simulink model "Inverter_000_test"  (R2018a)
settings: Solver=FixedStepDiscrete  StartTime=0.0  StopTime=inf  RelTol=1e-3  EnableMultiTasking=on
PreLoadFcn:
  | Sample_Time
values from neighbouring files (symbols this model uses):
  Tcontrol = 5e-5     *2    (= 0.0001)    [Sample_Time.m]
undefined symbols (not defined in the file or in its folder): A, ADCIN0, ADCIN1, ADCINA0, ADCINB0, bit, Compare, conversion, DCAEVT1, DCAEVT1FILT, Digital, Down, ended, Event, Filtered, GPTRIP1SEL, GPTRIP2SEL, input, Module, of, Single, start, Trip, TZ1, TZ2, Up, version, Zone
libraries: tiiqmathlib x19, c2837xDlib x6, c2802xlib x5, simulink x4, etargetslib x4, c28xdmclib x1

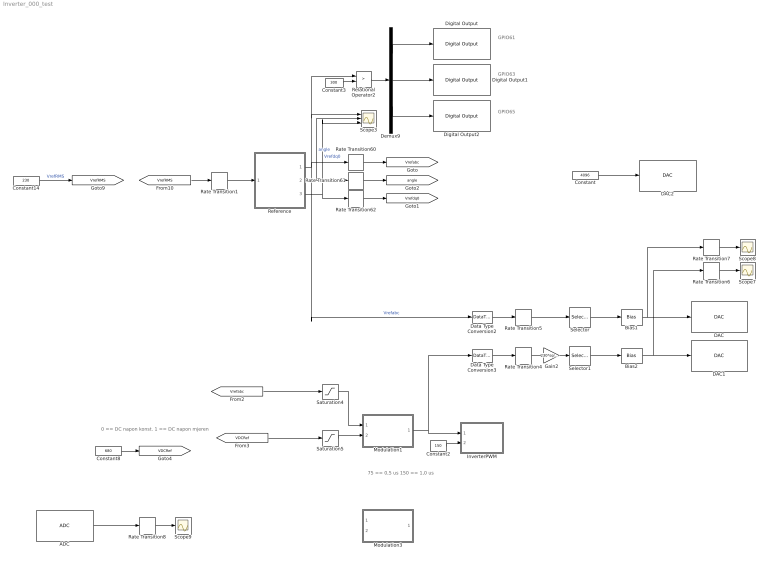
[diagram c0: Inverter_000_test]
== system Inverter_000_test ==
  note: 0 == DC napon konst. 1 == DC napon mjeren
  note: 75 == 0,5 us 150 == 1,0 us
  note: GPIO61
  note: GPIO63
  note: GPIO65
  ADC : c2802xlib/ADC  Commented=on  blkParamProc=C2000_Type4  ADCModule=B  samplingMode=Single sample mode  ADCResolution=12-bit (Single-ended input)  useSOC1=SOC0  useSOC2=SOC0_SOC1  SOCAcquisitionWindow=15  SOCTriggerSource=Software  SOCInterruptTrigger=ADCINT1  Ts=0.001  dType=uint16  postInterrupt=on  interruptSel=ADCINT1  ADCINTContinuous=on  endma=off  chdma=1  conv1=ADCINA0  conv2=ADCINA0 and ADCINB0  conv1_Type4=ADCIN2  conv2_Type4=ADCIN0 and ADCIN1
  Bias1 : Bias  Bias=400
  Bias2 : Bias  Bias=400
  Constant : Constant  Value=4096
  Constant14 : Constant  Value=230  OutDataTypeStr=single  SampleTime=Tcontrol
  Constant2 : Constant  Value=150  OutDataTypeStr=single
  Constant3 : Constant  Value=300  OutDataTypeStr=fixdt(1,32,2^-10,0)
  Constant8 : Constant  Value=680  OutDataTypeStr=fixdt(1,32,2^-10,0)
  DAC : c2837xDlib/DAC  channel=A  saturate=on
  DAC1 : c2837xDlib/DAC  channel=B  saturate=on
  DAC2 : c2837xDlib/DAC  channel=C  saturate=on
  Data Type Conversion2 : DataTypeConversion  OutDataTypeStr=single
  Data Type Conversion3 : DataTypeConversion  OutDataTypeStr=single
  Demux9 : Demux  Outputs=3
  Digital Output : c2837xDlib/Digital Output  GPIO_Number=GPIO56~GPIO63  GPIO_Bit0=off  GPIO_BIT0_Toggle=off  GPIO_Bit1=off  GPIO_BIT1_Toggle=off  GPIO_Bit2=off  GPIO_BIT2_Toggle=off  GPIO_Bit3=off  GPIO_BIT3_Toggle=off  GPIO_Bit4=off  GPIO_BIT4_Toggle=off  GPIO_Bit5=on  GPIO_BIT5_Toggle=off  GPIO_Bit6=off  GPIO_BIT6_Toggle=off  GPIO_Bit7=off  GPIO_BIT7_Toggle=off
  Digital Output1 : c2837xDlib/Digital Output  GPIO_Number=GPIO56~GPIO63  GPIO_Bit0=off  GPIO_BIT0_Toggle=off  GPIO_Bit1=off  GPIO_BIT1_Toggle=off  GPIO_Bit2=off  GPIO_BIT2_Toggle=off  GPIO_Bit3=off  GPIO_BIT3_Toggle=off  GPIO_Bit4=off  GPIO_BIT4_Toggle=off  GPIO_Bit5=off  GPIO_BIT5_Toggle=off  GPIO_Bit6=off  GPIO_BIT6_Toggle=off  GPIO_Bit7=on  GPIO_BIT7_Toggle=off
  Digital Output2 : c2837xDlib/Digital Output  GPIO_Number=GPIO64~GPIO71  GPIO_Bit0=off  GPIO_BIT0_Toggle=off  GPIO_Bit1=off  GPIO_BIT1_Toggle=off  GPIO_Bit2=on  GPIO_BIT2_Toggle=off  GPIO_Bit3=off  GPIO_BIT3_Toggle=off  GPIO_Bit4=off  GPIO_BIT4_Toggle=off  GPIO_Bit5=off  GPIO_BIT5_Toggle=off  GPIO_Bit6=off  GPIO_BIT6_Toggle=off  GPIO_Bit7=off  GPIO_BIT7_Toggle=off
  Gain2 : Gain  Gain=230*sqrt(2)
  InverterPWM : Subsystem
  Modulation1 : Subsystem
  Modulation3 : Subsystem  Commented=on
  Rate Transition1 : RateTransition  OutPortSampleTime=5e-5
  Rate Transition{4..5,60..62} (5 alike) : RateTransition  OutPortSampleTime=Tcontrol
  Rate Transition6 : RateTransition  Commented=on  OutPortSampleTime=5e-4
  Rate Transition7 : RateTransition  Commented=on  OutPortSampleTime=5e-4
  Rate Transition8 : RateTransition  Commented=on  OutPortSampleTime=5e-4
  Reference : Subsystem
  Relational Operator2 : RelationalOperator  Operator=>  OutDataTypeStr=boolean
  Saturation4 : Saturate  UpperLimit=400  LowerLimit=-400
  Saturation5 : Saturate  UpperLimit=720  LowerLimit=0
  Scope3 : Scope  NumInputPorts=3
  Scope7 : Scope
  Scope8 : Scope
  Scope9 : Scope
  Selector : Selector  InputPortWidth=3  IndexOptions=Index vector (dialog)  Indices=[2]  OutputSizes=1
  Selector1 : Selector  InputPortWidth=4  IndexOptions=Index vector (dialog)  Indices=[2]  OutputSizes=1
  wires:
  Constant8/1 -> [VDCRef]
  [Vrefabc] -> Saturation4/1
  Constant2/1 -> InverterPWM/2(DeadBand)
  Saturation4/1 -> Modulation1/1(Vcontrol)
  Modulation1/1(VPWM) -> InverterPWM/1(PWM), Data Type Conversion3/1
  Saturation5/1 -> Modulation1/2(VDC)
  [VDCRef] -> Saturation5/1
  Constant14/1 -> [VrefRMS]  "VrefRMS"
  Demux9/2 -> Digital Output1/1
  Rate Transition1/1 -> Reference/1(Vac Ref)
  [VrefRMS] -> Rate Transition1/1
  Rate Transition61/1 -> [angle]
  Reference/3(dq0) -> Scope3/3, Rate Transition62/1  "Vrefdq0"
  Rate Transition62/1 -> [Vrefdq0]
  Reference/1(abc) -> Data Type Conversion2/1, Scope3/1, Relational Operator2/1, Rate Transition60/1  "Vrefabc"
  Demux9/3 -> Digital Output2/1
  Reference/2(angle) -> Scope3/2, Rate Transition61/1  "angle"
  Rate Transition60/1 -> [Vrefabc]
  Demux9/1 -> Digital Output/1
  Relational Operator2/1 -> Demux9/1
  Constant3/1 -> Relational Operator2/2
  Rate Transition4/1 -> Gain2/1
  Rate Transition5/1 -> Selector/1
  Data Type Conversion2/1 -> Rate Transition5/1
  Data Type Conversion3/1 -> Rate Transition4/1
  Gain2/1 -> Selector1/1
  Selector/1 -> Bias1/1
  Selector1/1 -> Bias2/1
  Bias1/1 -> DAC/1, Rate Transition7/1
  Bias2/1 -> Rate Transition6/1, DAC1/1
  Rate Transition6/1 -> Scope7/1
  Rate Transition7/1 -> Scope8/1
  Constant/1 -> DAC2/1
  Rate Transition8/1 -> Scope9/1
  ADC/1 -> Rate Transition8/1

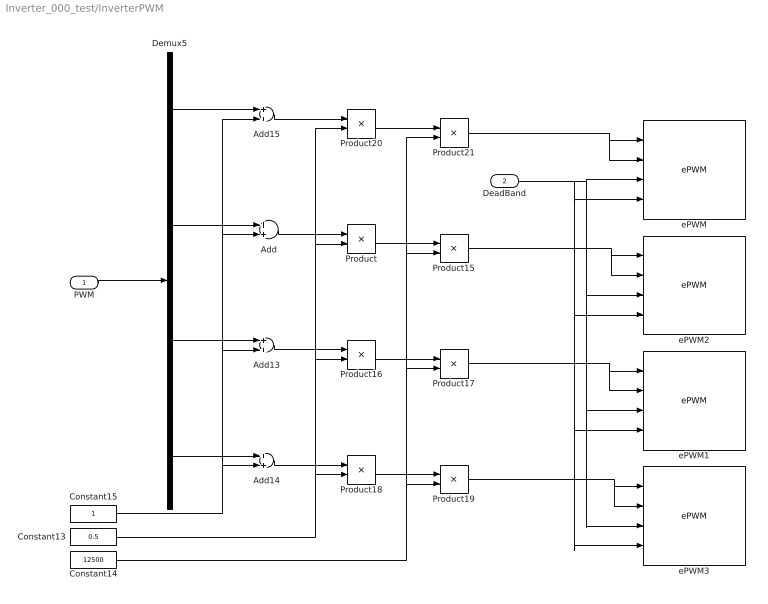
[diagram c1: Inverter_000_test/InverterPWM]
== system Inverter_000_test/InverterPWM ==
  PWM : Inport
  DeadBand : Inport  Port=2
  Add{,13..15} (4 alike) : Sum
  Constant13 : Constant  Value=0.5  OutDataTypeStr=single
  Constant14 : Constant  Value=12500  OutDataTypeStr=single
  Constant15 : Constant  OutDataTypeStr=single
  Demux5 : Demux
  Product{,15..21} (8 alike) : Product
  ePWM : c2802xlib/ePWM  useModule=ePWM5  ePWMxLINKTBPRD=Not Linked  periodUnits=Clock cycles  timerSource=Specify via dialog  timerPeriod_clk=12500  timerPeriod_sec=0.0001  tbshadow=Counter equals to zero  countingMode=Up-Down  phaseActiveEnable=Disable  phaseDirection=Count down after sync  phaseActive=0  synchronizationEnable=off  dcaevt1Sync=off  dcbevt1Sync=off  synchronizationOption=Disable  clockPrescale=1  HSclockPrescale=1  enswap=off  ePWMxAStatus=on  ePWMxAactionLogic1=Set  ePWMxAactionLogic2=Clear  ePWMxAactionLogic3=Clear  ePWMxAactionLogic4=Set  ePWMxAactionLogic5=Do nothing  ePWMxAactionLogic6=Do nothing  ePWMxALoadMode=Load on counter equals to zero (CTR=Zero)  ePWMxACSFenable=off  ePWMxACSFvalue=Forcing disable  ePWMxASFreload=Zero  ePWMxBStatus=on  ePWMxBactionLogic1=Clear  ePWMxBactionLogic2=Set  ePWMxBactionLogic3=Do nothing  ePWMxBactionLogic4=Do nothing  ePWMxBactionLogic5=Set  ePWMxBactionLogic6=Clear  ePWMxBLoadMode=Load on counter equals to zero (CTR=Zero)  ePWMxBCSFenable=off  ePWMxBCSFvalue=Forcing disable  ePWMxBSFreload=Zero  ePWNxBOutWay=off  ePWMxLINKCMPA=Not Linked  CMPAUnits=Clock cycles  CMPASource=Input port  CMPAValue_per=50  CMPAValue_clk=3750  enCMPAshadow=Counter equals to zero  ePWMxLINKCMPB=Not Linked  CMPBUnits=Clock cycles  CMPBSource=Input port  CMPBValue_per=50  CMPBValue_clk=3750  enCMPBshadow=Counter equals to zero  ePWMxLINKCMPC=Not Linked  CMPCUnits=Clock cycles  CMPCSource=Specify via dialog  CMPCValue_per=50  CMPCValue_clk=32000  enCMPCshadow=Counter equals to zero  ePWMxLINKCMPD=Not Linked  CMPDUnits=Clock cycles  CMPDSource=Specify via dialog  CMPDValue_per=50  CMPDValue_clk=32000  enCMPDshadow=Counter equals to zero  enableDBePWMxA=on  enableDBePWMxB=on  enhalfcycle=off  DBpolarity=Active high complementary (AHC)  DBedgeDelay=Positive  DBSource_ePWMxA=ePWMxA  DBSource_ePWMxB=ePWMxA  DBperiodSource=Input port  REDperiod=0  FEDperiod=0  adcstartModuleA=off  adcrequestEventA=First event  adcstartEventA=Digital Compare Module A Event 1 start of conversion (DCAEVT1.soc)  adcstartEventA_type2=Digital Compare Module A Event 1 start of conversion (DCAEVT1.soc)  adcstartModuleB=off  adcrequestEventB=First event  adcstartEventB=Counter equals to zero (CTR=Zero)  adcstartEventB_type2=Counter equals to zero (CTR=Zero)  intEn=off  intPrd=First event  intSel=Counter equals to zero (CTR=Zero)  intSel_type2=Counter equals to zero (CTR=Zero)  hrpe=off  enHRPWM=off  HRPWM_LoadMode=Counter equals to period (CTR=PRD)  HRPWM_CTLMode=Duty or Period control mode  HRPWM_EDGMode=Both edge  hrpeb=off  enHRPWMB=off  HRPWM_LoadModeB=Counter equals to zero (CTR=ZERO)  HRPWM_CTLModeB=Duty or Period control mode  HRPWM_EDGModeB=Both edge  enSFO=on  enautoconv=on  chopperEnable=off  chopperFrequency=1  chopperFirstwidth=1  chopperDuty=12.5%  tripZonesource=Specify via dialog  tzselOSHT1=off  tzselOSHT2=off  tzselOSHT3=off  tzselOSHDCAEV1=off  tzselOSHDCBEV1=off  tzselCBC1=off  tzselCBC2=off  tzselCBC3=off  tzselCBCDCAEV2=off  tzselCBCDCBEV2=off  tzselOSHT4=off  tzselOSHT5=off  tzselOSHT6=off  tzselCBC4=off  tzselCBC5=off  tzselCBC6=off  enTzOstIntr=off  enTzCbcIntr=off  enTzDCAEVT1Intr=off  enTzDCAEVT2Intr=off  enTzDCBEVT1Intr=off  enTzDCBEVT2Intr=off  ePWMxAforced=No action  ePWMxBforced=No action  DCAEVT1forced=No action  DCBEVT1forced=No action  DCAEVT2forced=No action  DCBEVT2forced=No action  dcah=Trip Zone 1 input (TZ1)  dcal=Trip Zone 2 input (TZ2)  dcbh=Trip Zone 1 input (TZ1)  dcbl=Trip Zone 2 input (TZ2)  dcah_type2=GPTRIP1SEL/(TZ1)  dcal_type2=GPTRIP2SEL/(TZ2)  dcbh_type2=GPTRIP1SEL/(TZ1)  dcbl_type2=GPTRIP2SEL/(TZ2)  gendcaevt1=Event disabled  gendcaevt2=Event disabled  gendcbevt1=Event disabled  gendcbevt2=Event disabled  dcaevt1src=DCAEVT1 with sync  dcaevt2src=DCAEVT2 with sync  dcbevt1src=DCBEVT1 with sync  dcbevt2src=DCBEVT2 with sync  pulsesel=Counter equals to zero (CTR=Zero)  blankinv=off  blankoffset=0  blankwidth=0  evsrcsel=Filtered version of DCAEVT1 (DCAEVT1FILT)  encape=off  PwmType=C2000_Type4
  ePWM1 : c2802xlib/ePWM  useModule=ePWM3  ePWMxLINKTBPRD=Not Linked  periodUnits=Clock cycles  timerSource=Specify via dialog  timerPeriod_clk=12500  timerPeriod_sec=0.0001  tbshadow=Counter equals to zero  countingMode=Up-Down  phaseActiveEnable=Disable  phaseDirection=Count down after sync  phaseActive=0  synchronizationEnable=off  dcaevt1Sync=off  dcbevt1Sync=off  synchronizationOption=Disable  clockPrescale=1  HSclockPrescale=1  enswap=off  ePWMxAStatus=on  ePWMxAactionLogic1=Set  ePWMxAactionLogic2=Clear  ePWMxAactionLogic3=Clear  ePWMxAactionLogic4=Set  ePWMxAactionLogic5=Do nothing  ePWMxAactionLogic6=Do nothing  ePWMxALoadMode=Load on counter equals to zero (CTR=Zero)  ePWMxACSFenable=off  ePWMxACSFvalue=Forcing disable  ePWMxASFreload=Zero  ePWMxBStatus=on  ePWMxBactionLogic1=Clear  ePWMxBactionLogic2=Set  ePWMxBactionLogic3=Do nothing  ePWMxBactionLogic4=Do nothing  ePWMxBactionLogic5=Set  ePWMxBactionLogic6=Clear  ePWMxBLoadMode=Load on counter equals to zero (CTR=Zero)  ePWMxBCSFenable=off  ePWMxBCSFvalue=Forcing disable  ePWMxBSFreload=Zero  ePWNxBOutWay=off  ePWMxLINKCMPA=Not Linked  CMPAUnits=Clock cycles  CMPASource=Input port  CMPAValue_per=50  CMPAValue_clk=3750  enCMPAshadow=Counter equals to zero  ePWMxLINKCMPB=Not Linked  CMPBUnits=Clock cycles  CMPBSource=Input port  CMPBValue_per=50  CMPBValue_clk=3750  enCMPBshadow=Counter equals to zero  ePWMxLINKCMPC=Not Linked  CMPCUnits=Clock cycles  CMPCSource=Specify via dialog  CMPCValue_per=50  CMPCValue_clk=32000  enCMPCshadow=Counter equals to zero  ePWMxLINKCMPD=Not Linked  CMPDUnits=Clock cycles  CMPDSource=Specify via dialog  CMPDValue_per=50  CMPDValue_clk=32000  enCMPDshadow=Counter equals to zero  enableDBePWMxA=on  enableDBePWMxB=on  enhalfcycle=off  DBpolarity=Active high complementary (AHC)  DBedgeDelay=Positive  DBSource_ePWMxA=ePWMxA  DBSource_ePWMxB=ePWMxA  DBperiodSource=Input port  REDperiod=0  FEDperiod=0  adcstartModuleA=off  adcrequestEventA=First event  adcstartEventA=Digital Compare Module A Event 1 start of conversion (DCAEVT1.soc)  adcstartEventA_type2=Digital Compare Module A Event 1 start of conversion (DCAEVT1.soc)  adcstartModuleB=off  adcrequestEventB=First event  adcstartEventB=Counter equals to zero (CTR=Zero)  adcstartEventB_type2=Counter equals to zero (CTR=Zero)  intEn=off  intPrd=First event  intSel=Counter equals to zero (CTR=Zero)  intSel_type2=Counter equals to zero (CTR=Zero)  hrpe=off  enHRPWM=off  HRPWM_LoadMode=Counter equals to period (CTR=PRD)  HRPWM_CTLMode=Duty or Period control mode  HRPWM_EDGMode=Both edge  hrpeb=off  enHRPWMB=off  HRPWM_LoadModeB=Counter equals to zero (CTR=ZERO)  HRPWM_CTLModeB=Duty or Period control mode  HRPWM_EDGModeB=Both edge  enSFO=on  enautoconv=on  chopperEnable=off  chopperFrequency=1  chopperFirstwidth=1  chopperDuty=12.5%  tripZonesource=Specify via dialog  tzselOSHT1=off  tzselOSHT2=off  tzselOSHT3=off  tzselOSHDCAEV1=off  tzselOSHDCBEV1=off  tzselCBC1=off  tzselCBC2=off  tzselCBC3=off  tzselCBCDCAEV2=off  tzselCBCDCBEV2=off  tzselOSHT4=off  tzselOSHT5=off  tzselOSHT6=off  tzselCBC4=off  tzselCBC5=off  tzselCBC6=off  enTzOstIntr=off  enTzCbcIntr=off  enTzDCAEVT1Intr=off  enTzDCAEVT2Intr=off  enTzDCBEVT1Intr=off  enTzDCBEVT2Intr=off  ePWMxAforced=No action  ePWMxBforced=No action  DCAEVT1forced=No action  DCBEVT1forced=No action  DCAEVT2forced=No action  DCBEVT2forced=No action  dcah=Trip Zone 1 input (TZ1)  dcal=Trip Zone 2 input (TZ2)  dcbh=Trip Zone 1 input (TZ1)  dcbl=Trip Zone 2 input (TZ2)  dcah_type2=GPTRIP1SEL/(TZ1)  dcal_type2=GPTRIP2SEL/(TZ2)  dcbh_type2=GPTRIP1SEL/(TZ1)  dcbl_type2=GPTRIP2SEL/(TZ2)  gendcaevt1=Event disabled  gendcaevt2=Event disabled  gendcbevt1=Event disabled  gendcbevt2=Event disabled  dcaevt1src=DCAEVT1 with sync  dcaevt2src=DCAEVT2 with sync  dcbevt1src=DCBEVT1 with sync  dcbevt2src=DCBEVT2 with sync  pulsesel=Counter equals to zero (CTR=Zero)  blankinv=off  blankoffset=0  blankwidth=0  evsrcsel=Filtered version of DCAEVT1 (DCAEVT1FILT)  encape=off  PwmType=C2000_Type4
  ePWM2 : c2802xlib/ePWM  useModule=ePWM6  ePWMxLINKTBPRD=Not Linked  periodUnits=Clock cycles  timerSource=Specify via dialog  timerPeriod_clk=12500  timerPeriod_sec=0.0001  tbshadow=Counter equals to zero  countingMode=Up-Down  phaseActiveEnable=Disable  phaseDirection=Count down after sync  phaseActive=0  synchronizationEnable=off  dcaevt1Sync=off  dcbevt1Sync=off  synchronizationOption=Disable  clockPrescale=1  HSclockPrescale=1  enswap=off  ePWMxAStatus=on  ePWMxAactionLogic1=Set  ePWMxAactionLogic2=Clear  ePWMxAactionLogic3=Clear  ePWMxAactionLogic4=Set  ePWMxAactionLogic5=Do nothing  ePWMxAactionLogic6=Do nothing  ePWMxALoadMode=Load on counter equals to zero (CTR=Zero)  ePWMxACSFenable=off  ePWMxACSFvalue=Forcing disable  ePWMxASFreload=Zero  ePWMxBStatus=on  ePWMxBactionLogic1=Clear  ePWMxBactionLogic2=Set  ePWMxBactionLogic3=Do nothing  ePWMxBactionLogic4=Do nothing  ePWMxBactionLogic5=Set  ePWMxBactionLogic6=Clear  ePWMxBLoadMode=Load on counter equals to zero (CTR=Zero)  ePWMxBCSFenable=off  ePWMxBCSFvalue=Forcing disable  ePWMxBSFreload=Zero  ePWNxBOutWay=off  ePWMxLINKCMPA=Not Linked  CMPAUnits=Clock cycles  CMPASource=Input port  CMPAValue_per=50  CMPAValue_clk=3750  enCMPAshadow=Counter equals to zero  ePWMxLINKCMPB=Not Linked  CMPBUnits=Clock cycles  CMPBSource=Input port  CMPBValue_per=50  CMPBValue_clk=3750  enCMPBshadow=Counter equals to zero  ePWMxLINKCMPC=Not Linked  CMPCUnits=Clock cycles  CMPCSource=Specify via dialog  CMPCValue_per=50  CMPCValue_clk=32000  enCMPCshadow=Counter equals to zero  ePWMxLINKCMPD=Not Linked  CMPDUnits=Clock cycles  CMPDSource=Specify via dialog  CMPDValue_per=50  CMPDValue_clk=32000  enCMPDshadow=Counter equals to zero  enableDBePWMxA=on  enableDBePWMxB=on  enhalfcycle=off  DBpolarity=Active high complementary (AHC)  DBedgeDelay=Positive  DBSource_ePWMxA=ePWMxA  DBSource_ePWMxB=ePWMxA  DBperiodSource=Input port  REDperiod=0  FEDperiod=0  adcstartModuleA=off  adcrequestEventA=First event  adcstartEventA=Digital Compare Module A Event 1 start of conversion (DCAEVT1.soc)  adcstartEventA_type2=Digital Compare Module A Event 1 start of conversion (DCAEVT1.soc)  adcstartModuleB=off  adcrequestEventB=First event  adcstartEventB=Counter equals to zero (CTR=Zero)  adcstartEventB_type2=Counter equals to zero (CTR=Zero)  intEn=off  intPrd=First event  intSel=Counter equals to zero (CTR=Zero)  intSel_type2=Counter equals to zero (CTR=Zero)  hrpe=off  enHRPWM=off  HRPWM_LoadMode=Counter equals to period (CTR=PRD)  HRPWM_CTLMode=Duty or Period control mode  HRPWM_EDGMode=Both edge  hrpeb=off  enHRPWMB=off  HRPWM_LoadModeB=Counter equals to zero (CTR=ZERO)  HRPWM_CTLModeB=Duty or Period control mode  HRPWM_EDGModeB=Both edge  enSFO=on  enautoconv=on  chopperEnable=off  chopperFrequency=1  chopperFirstwidth=1  chopperDuty=12.5%  tripZonesource=Specify via dialog  tzselOSHT1=off  tzselOSHT2=off  tzselOSHT3=off  tzselOSHDCAEV1=off  tzselOSHDCBEV1=off  tzselCBC1=off  tzselCBC2=off  tzselCBC3=off  tzselCBCDCAEV2=off  tzselCBCDCBEV2=off  tzselOSHT4=off  tzselOSHT5=off  tzselOSHT6=off  tzselCBC4=off  tzselCBC5=off  tzselCBC6=off  enTzOstIntr=off  enTzCbcIntr=off  enTzDCAEVT1Intr=off  enTzDCAEVT2Intr=off  enTzDCBEVT1Intr=off  enTzDCBEVT2Intr=off  ePWMxAforced=No action  ePWMxBforced=No action  DCAEVT1forced=No action  DCBEVT1forced=No action  DCAEVT2forced=No action  DCBEVT2forced=No action  dcah=Trip Zone 1 input (TZ1)  dcal=Trip Zone 2 input (TZ2)  dcbh=Trip Zone 1 input (TZ1)  dcbl=Trip Zone 2 input (TZ2)  dcah_type2=GPTRIP1SEL/(TZ1)  dcal_type2=GPTRIP2SEL/(TZ2)  dcbh_type2=GPTRIP1SEL/(TZ1)  dcbl_type2=GPTRIP2SEL/(TZ2)  gendcaevt1=Event disabled  gendcaevt2=Event disabled  gendcbevt1=Event disabled  gendcbevt2=Event disabled  dcaevt1src=DCAEVT1 with sync  dcaevt2src=DCAEVT2 with sync  dcbevt1src=DCBEVT1 with sync  dcbevt2src=DCBEVT2 with sync  pulsesel=Counter equals to zero (CTR=Zero)  blankinv=off  blankoffset=0  blankwidth=0  evsrcsel=Filtered version of DCAEVT1 (DCAEVT1FILT)  encape=off  PwmType=C2000_Type4
  ePWM3 : c2802xlib/ePWM  useModule=ePWM4  ePWMxLINKTBPRD=Not Linked  periodUnits=Clock cycles  timerSource=Specify via dialog  timerPeriod_clk=12500  timerPeriod_sec=0.0001  tbshadow=Counter equals to zero  countingMode=Up-Down  phaseActiveEnable=Disable  phaseDirection=Count down after sync  phaseActive=0  synchronizationEnable=off  dcaevt1Sync=off  dcbevt1Sync=off  synchronizationOption=Disable  clockPrescale=1  HSclockPrescale=1  enswap=off  ePWMxAStatus=on  ePWMxAactionLogic1=Set  ePWMxAactionLogic2=Clear  ePWMxAactionLogic3=Clear  ePWMxAactionLogic4=Set  ePWMxAactionLogic5=Do nothing  ePWMxAactionLogic6=Do nothing  ePWMxALoadMode=Load on counter equals to zero (CTR=Zero)  ePWMxACSFenable=off  ePWMxACSFvalue=Forcing disable  ePWMxASFreload=Zero  ePWMxBStatus=on  ePWMxBactionLogic1=Clear  ePWMxBactionLogic2=Set  ePWMxBactionLogic3=Do nothing  ePWMxBactionLogic4=Do nothing  ePWMxBactionLogic5=Set  ePWMxBactionLogic6=Clear  ePWMxBLoadMode=Load on counter equals to zero (CTR=Zero)  ePWMxBCSFenable=off  ePWMxBCSFvalue=Forcing disable  ePWMxBSFreload=Zero  ePWNxBOutWay=off  ePWMxLINKCMPA=Not Linked  CMPAUnits=Clock cycles  CMPASource=Input port  CMPAValue_per=50  CMPAValue_clk=3750  enCMPAshadow=Counter equals to zero  ePWMxLINKCMPB=Not Linked  CMPBUnits=Clock cycles  CMPBSource=Input port  CMPBValue_per=50  CMPBValue_clk=3750  enCMPBshadow=Counter equals to zero  ePWMxLINKCMPC=Not Linked  CMPCUnits=Clock cycles  CMPCSource=Specify via dialog  CMPCValue_per=50  CMPCValue_clk=32000  enCMPCshadow=Counter equals to zero  ePWMxLINKCMPD=Not Linked  CMPDUnits=Clock cycles  CMPDSource=Specify via dialog  CMPDValue_per=50  CMPDValue_clk=32000  enCMPDshadow=Counter equals to zero  enableDBePWMxA=on  enableDBePWMxB=on  enhalfcycle=off  DBpolarity=Active high complementary (AHC)  DBedgeDelay=Positive  DBSource_ePWMxA=ePWMxA  DBSource_ePWMxB=ePWMxA  DBperiodSource=Input port  REDperiod=0  FEDperiod=0  adcstartModuleA=off  adcrequestEventA=First event  adcstartEventA=Digital Compare Module A Event 1 start of conversion (DCAEVT1.soc)  adcstartEventA_type2=Digital Compare Module A Event 1 start of conversion (DCAEVT1.soc)  adcstartModuleB=off  adcrequestEventB=First event  adcstartEventB=Counter equals to zero (CTR=Zero)  adcstartEventB_type2=Counter equals to zero (CTR=Zero)  intEn=off  intPrd=First event  intSel=Counter equals to zero (CTR=Zero)  intSel_type2=Counter equals to zero (CTR=Zero)  hrpe=off  enHRPWM=off  HRPWM_LoadMode=Counter equals to period (CTR=PRD)  HRPWM_CTLMode=Duty or Period control mode  HRPWM_EDGMode=Both edge  hrpeb=off  enHRPWMB=off  HRPWM_LoadModeB=Counter equals to zero (CTR=ZERO)  HRPWM_CTLModeB=Duty or Period control mode  HRPWM_EDGModeB=Both edge  enSFO=on  enautoconv=on  chopperEnable=off  chopperFrequency=1  chopperFirstwidth=1  chopperDuty=12.5%  tripZonesource=Specify via dialog  tzselOSHT1=off  tzselOSHT2=off  tzselOSHT3=off  tzselOSHDCAEV1=off  tzselOSHDCBEV1=off  tzselCBC1=off  tzselCBC2=off  tzselCBC3=off  tzselCBCDCAEV2=off  tzselCBCDCBEV2=off  tzselOSHT4=off  tzselOSHT5=off  tzselOSHT6=off  tzselCBC4=off  tzselCBC5=off  tzselCBC6=off  enTzOstIntr=off  enTzCbcIntr=off  enTzDCAEVT1Intr=off  enTzDCAEVT2Intr=off  enTzDCBEVT1Intr=off  enTzDCBEVT2Intr=off  ePWMxAforced=No action  ePWMxBforced=No action  DCAEVT1forced=No action  DCBEVT1forced=No action  DCAEVT2forced=No action  DCBEVT2forced=No action  dcah=Trip Zone 1 input (TZ1)  dcal=Trip Zone 2 input (TZ2)  dcbh=Trip Zone 1 input (TZ1)  dcbl=Trip Zone 2 input (TZ2)  dcah_type2=GPTRIP1SEL/(TZ1)  dcal_type2=GPTRIP2SEL/(TZ2)  dcbh_type2=GPTRIP1SEL/(TZ1)  dcbl_type2=GPTRIP2SEL/(TZ2)  gendcaevt1=Event disabled  gendcaevt2=Event disabled  gendcbevt1=Event disabled  gendcbevt2=Event disabled  dcaevt1src=DCAEVT1 with sync  dcaevt2src=DCAEVT2 with sync  dcbevt1src=DCBEVT1 with sync  dcbevt2src=DCBEVT2 with sync  pulsesel=Counter equals to zero (CTR=Zero)  blankinv=off  blankoffset=0  blankwidth=0  evsrcsel=Filtered version of DCAEVT1 (DCAEVT1FILT)  encape=off  PwmType=C2000_Type4
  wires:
  PWM/1 -> Demux5/1
  Product/1 -> Product15/1
  Add/1 -> Product/1
  Add14/1 -> Product18/1
  Add13/1 -> Product16/1
  Product18/1 -> Product19/1
  Product16/1 -> Product17/1
  Constant15/1 -> Add15/2, Add/2, Add13/2, Add14/2
  Product20/1 -> Product21/1
  Add15/1 -> Product20/1
  Constant14/1 -> Product17/2, Product21/2, Product15/2, Product19/2
  Constant13/1 -> Product18/2, Product16/2, Product20/2, Product/2
  Demux5/1 -> Add15/1
  Demux5/2 -> Add/1
  Demux5/3 -> Add13/1
  Demux5/4 -> Add14/1
  Product19/1 -> ePWM3/1, ePWM3/2
  Product15/1 -> ePWM2/1, ePWM2/2
  Product17/1 -> ePWM1/1, ePWM1/2
  Product21/1 -> ePWM/1, ePWM/2
  DeadBand/1 -> ePWM/4, ePWM2/4, ePWM3/4, ePWM1/4, ePWM/3, ePWM2/3, ePWM3/3, ePWM1/3

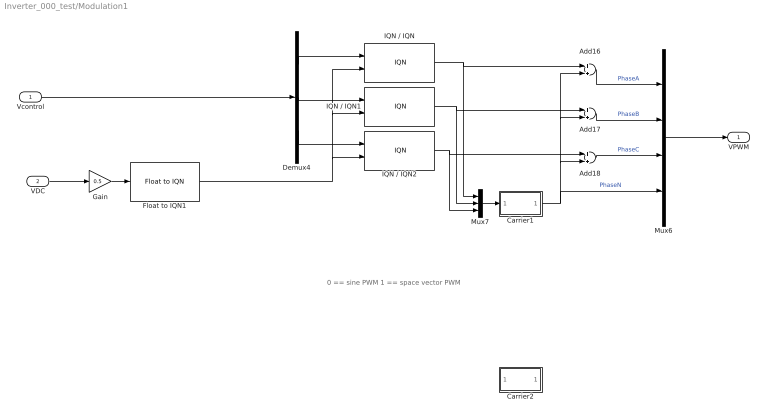
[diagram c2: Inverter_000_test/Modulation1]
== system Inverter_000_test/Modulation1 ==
  note: 0 == sine PWM 1 == space vector PWM
  Vcontrol : Inport
  VDC : Inport  Port=2
  Add16 : Sum
  Add17 : Sum
  Add18 : Sum
  Carrier1 : Subsystem
  Carrier2 : Subsystem  Commented=on
  Demux4 : Demux  Outputs=3
  Float to IQN1 : tiiqmathlib/Float to IQN  Q_value=10
  Gain : Gain  Gain=0.5  OutDataTypeStr=single
  IQN / IQN : tiiqmathlib/IQN // IQN
  IQN / IQN1 : tiiqmathlib/IQN // IQN
  IQN / IQN2 : tiiqmathlib/IQN // IQN
  Mux6 : Mux
  Mux7 : Mux  Inputs=3
  VPWM : Outport
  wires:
  Add17/1 -> Mux6/2  "PhaseB"
  Carrier1/1(Out1) -> Mux6/4, Add16/2, Add17/2, Add18/2  "PhaseN"
  Demux4/2 -> IQN / IQN1/1
  Add16/1 -> Mux6/1  "PhaseA"
  Mux7/1 -> Carrier1/1(In1)
  IQN / IQN1/1 -> Mux7/2, Add17/1
  Demux4/1 -> IQN / IQN/1
  Mux6/1 -> VPWM/1
  Demux4/3 -> IQN / IQN2/1
  VDC/1 -> Gain/1
  Add18/1 -> Mux6/3  "PhaseC"
  IQN / IQN2/1 -> Mux7/3, Add18/1
  Gain/1 -> Float to IQN1/1
  Vcontrol/1 -> Demux4/1
  Float to IQN1/1 -> IQN / IQN1/2, IQN / IQN/2, IQN / IQN2/2
  IQN / IQN/1 -> Mux7/1, Add16/1

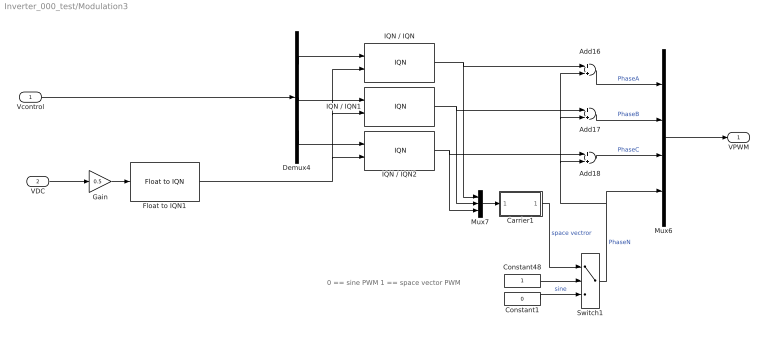
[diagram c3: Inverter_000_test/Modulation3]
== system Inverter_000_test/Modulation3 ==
  note: 0 == sine PWM 1 == space vector PWM
  Vcontrol : Inport
  VDC : Inport  Port=2
  Add16 : Sum
  Add17 : Sum
  Add18 : Sum
  Carrier1 : Subsystem
  Constant1 : Constant  Value=0  OutDataTypeStr=boolean
  Constant48 : Constant  OutDataTypeStr=boolean
  Demux4 : Demux  Outputs=3
  Float to IQN1 : tiiqmathlib/Float to IQN  Q_value=10
  Gain : Gain  Gain=0.5  OutDataTypeStr=single
  IQN / IQN : tiiqmathlib/IQN // IQN
  IQN / IQN1 : tiiqmathlib/IQN // IQN
  IQN / IQN2 : tiiqmathlib/IQN // IQN
  Mux6 : Mux
  Mux7 : Mux  Inputs=3
  Switch1 : Switch  Threshold=0.5
  VPWM : Outport
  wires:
  Float to IQN1/1 -> IQN / IQN2/2, IQN / IQN/2, IQN / IQN1/2
  Vcontrol/1 -> Demux4/1
  Gain/1 -> Float to IQN1/1
  IQN / IQN2/1 -> Add18/1, Mux7/3
  Add18/1 -> Mux6/3  "PhaseC"
  VDC/1 -> Gain/1
  Demux4/3 -> IQN / IQN2/1
  Mux6/1 -> VPWM/1
  Demux4/1 -> IQN / IQN/1
  IQN / IQN1/1 -> Add17/1, Mux7/2
  Mux7/1 -> Carrier1/1(In1)
  IQN / IQN/1 -> Add16/1, Mux7/1
  Add16/1 -> Mux6/1  "PhaseA"
  Demux4/2 -> IQN / IQN1/1
  Switch1/1 -> Mux6/4, Add18/2, Add17/2, Add16/2  "PhaseN"
  Add17/1 -> Mux6/2  "PhaseB"
  Constant48/1 -> Switch1/2
  Constant1/1 -> Switch1/3  "sine"
  Carrier1/1(Out1) -> Switch1/1  "space vectror"

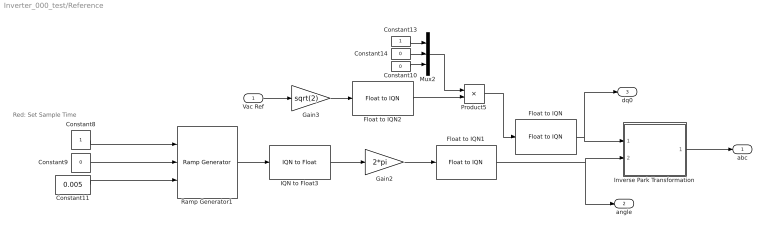
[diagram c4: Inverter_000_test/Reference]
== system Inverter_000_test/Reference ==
  note: Red: Set Sample Time
  Vac Ref : Inport
  Constant10 : Constant  Value=0  OutDataTypeStr=single
  Constant11 : Constant  Value=0.005  OutDataTypeStr=fixdt(1,32,2^-29,0)
  Constant13 : Constant  OutDataTypeStr=single
  Constant14 : Constant  Value=0  OutDataTypeStr=single
  Constant8 : Constant  OutDataTypeStr=fixdt(1,32,2^-29,0)  SampleTime=-1
  Constant9 : Constant  Value=0  OutDataTypeStr=fixdt(1,32,2^-29,0)
  Float to IQN : tiiqmathlib/Float to IQN  Q_value=10
  Float to IQN1 : tiiqmathlib/Float to IQN  Q_value=10
  Float to IQN2 : tiiqmathlib/Float to IQN  Q_value=10
  Gain2 : Gain  Gain=2*pi
  Gain3 : Gain  Gain=sqrt(2)  OutDataTypeStr=Inherit: Inherit via back propagation
  IQN to Float3 : tiiqmathlib/IQN to Float
  Inverse Park Transformation : Subsystem  InitFcn=tic2000lib_licenseCheck  mask(Inverse Park Transformation){}
      mask help: This block performs vector transformation from orthogonal rotating reference frame into orthogonal stationary frame. All inputs and outputs are signed 32-bit fixed-point numbers with Q value between 1 and 29.
  Mux2 : Mux  Inputs=3
  Product5 : Product
  Ramp Generator1 : c28xdmclib/Ramp Generator  step_angle_max=1
  abc : Outport
  angle : Outport  Port=2
  dq0 : Outport  Port=3
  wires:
  Vac Ref/1 -> Gain3/1
  IQN to Float3/1 -> Gain2/1
  Constant11/1 -> Ramp Generator1/3
  Gain2/1 -> Float to IQN1/1
  Constant14/1 -> Mux2/2
  Constant9/1 -> Ramp Generator1/2
  Float to IQN2/1 -> Product5/2
  Constant10/1 -> Mux2/3
  Product5/1 -> Float to IQN/1
  Constant13/1 -> Mux2/1
  Mux2/1 -> Product5/1
  Float to IQN1/1 -> angle/1, Inverse Park Transformation/2(theta)
  Constant8/1 -> Ramp Generator1/1
  Float to IQN/1 -> dq0/1, Inverse Park Transformation/1(DQ0)
  Gain3/1 -> Float to IQN2/1
  Ramp Generator1/1 -> IQN to Float3/1
  Inverse Park Transformation/1(ABC) -> abc/1

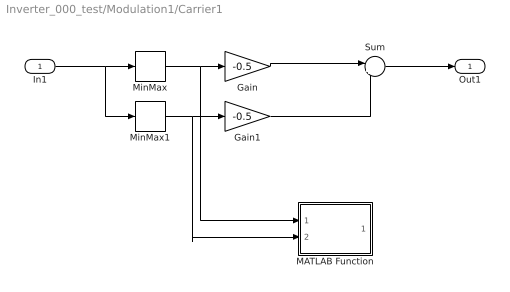
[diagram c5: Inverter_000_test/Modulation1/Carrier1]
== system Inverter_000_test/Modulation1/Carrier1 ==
  In1 : Inport
  Gain : Gain  Gain=-0.5
  Gain1 : Gain  Gain=-0.5
  MATLAB Function : MATLAB Function  Commented=on  TreatAsAtomicUnit=on
  MinMax : MinMax  ZeroCross=off
  MinMax1 : MinMax  Function=max  ZeroCross=off
  Sum : Sum  Inputs=|++
  Out1 : Outport
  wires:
  MinMax/1 -> MATLAB Function/1(In1), Gain/1
  MinMax1/1 -> MATLAB Function/2(In2), Gain1/1
  Gain/1 -> Sum/1
  Gain1/1 -> Sum/2
  In1/1 -> MinMax/1, MinMax1/1
  Sum/1 -> Out1/1

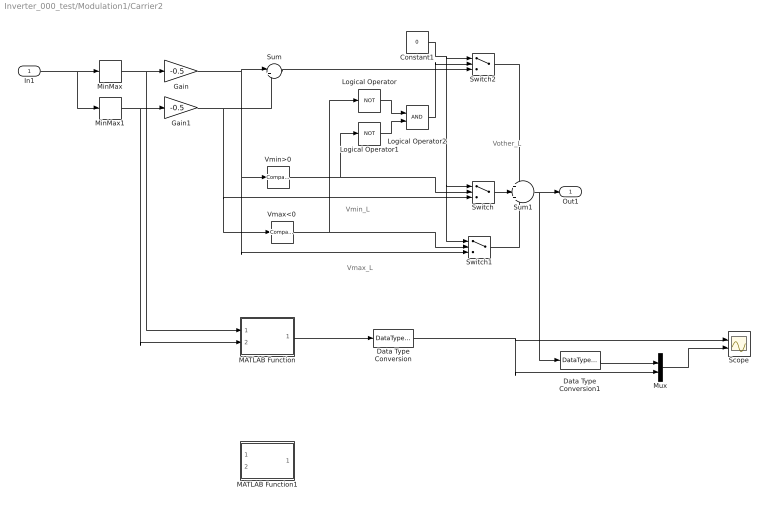
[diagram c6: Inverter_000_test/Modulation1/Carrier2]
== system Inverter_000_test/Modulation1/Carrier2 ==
  note: Vmax_L
  note: Vother_L
  note: Vmin_L
  In1 : Inport
  Constant1 : Constant  Value=0
  Data Type Conversion : DataTypeConversion  OutDataTypeStr=single
  Data Type Conversion1 : DataTypeConversion  OutDataTypeStr=single
  Gain : Gain  Gain=-0.5
  Gain1 : Gain  Gain=-0.5
  Logical Operator : Logic  Operator=NOT  AllPortsSameDT=off  OutDataTypeStr=boolean
  Logical Operator1 : Logic  Operator=NOT  AllPortsSameDT=off  OutDataTypeStr=boolean
  Logical Operator2 : Logic  AllPortsSameDT=off  OutDataTypeStr=boolean
  MATLAB Function : MATLAB Function  TreatAsAtomicUnit=on
  MATLAB Function1 : MATLAB Function  Commented=on  TreatAsAtomicUnit=on
  MinMax : MinMax  ZeroCross=off
  MinMax1 : MinMax  Function=max  ZeroCross=off
  Mux : Mux  Inputs=2
  Scope : Scope  NumInputPorts=2
  Sum : Sum  Inputs=|++
  Sum1 : Sum  Inputs=+|+|+
  Switch : Switch  Threshold=1  ZeroCross=off
  Switch1 : Switch  Threshold=1  ZeroCross=off
  Switch2 : Switch  Threshold=1  ZeroCross=off
  Vmax<0 : simulink/Logic and Bit Operations/Compare To Zero  relop=<  OutDataTypeStr=boolean  ZeroCross=off
  Vmin>0 : simulink/Logic and Bit Operations/Compare To Zero  relop=>  OutDataTypeStr=boolean  ZeroCross=off
  Out1 : Outport
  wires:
  Data Type Conversion1/1 -> Mux/1
  Data Type Conversion/1 -> Scope/1, Mux/2
  Mux/1 -> Scope/2
  MATLAB Function/1(y) -> Data Type Conversion/1
  Switch2/1 -> Sum1/1
  Switch/1 -> Sum1/2
  Constant1/1 -> Switch1/1, Switch/1, Switch2/1
  Sum1/1 -> Out1/1, Data Type Conversion1/1
  In1/1 -> MinMax1/1, MinMax/1
  Switch1/1 -> Sum1/3
  Sum/1 -> Switch2/3
  Logical Operator2/1 -> Switch2/2
  Vmax<0/1 -> Logical Operator/1, Switch1/2
  Vmin>0/1 -> Logical Operator1/1, Switch/2
  Logical Operator1/1 -> Logical Operator2/2
  Logical Operator/1 -> Logical Operator2/1
  Gain1/1 -> Sum/2, Switch/3, Vmax<0/1
  Gain/1 -> Sum/1, Vmin>0/1, Switch1/3
  MinMax1/1 -> Gain1/1, MATLAB Function/2(In2)
  MinMax/1 -> Gain/1, MATLAB Function/1(In1)

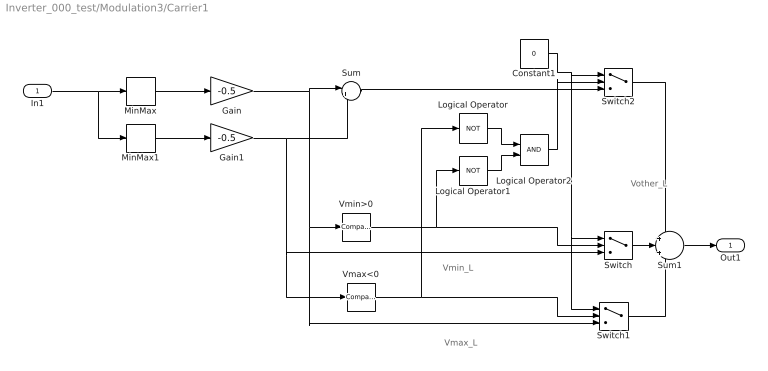
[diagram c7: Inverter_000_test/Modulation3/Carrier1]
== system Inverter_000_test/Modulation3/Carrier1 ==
  note: Vmax_L
  note: Vother_L
  note: Vmin_L
  In1 : Inport
  Constant1 : Constant  Value=0
  Gain : Gain  Gain=-0.5
  Gain1 : Gain  Gain=-0.5
  Logical Operator : Logic  Operator=NOT  AllPortsSameDT=off  OutDataTypeStr=boolean
  Logical Operator1 : Logic  Operator=NOT  AllPortsSameDT=off  OutDataTypeStr=boolean
  Logical Operator2 : Logic  AllPortsSameDT=off  OutDataTypeStr=boolean
  MinMax : MinMax  ZeroCross=off
  MinMax1 : MinMax  Function=max  ZeroCross=off
  Sum : Sum  Inputs=|++
  Sum1 : Sum  Inputs=+|+|+
  Switch : Switch  Threshold=1  ZeroCross=off
  Switch1 : Switch  Threshold=1  ZeroCross=off
  Switch2 : Switch  Threshold=1  ZeroCross=off
  Vmax<0 : simulink/Logic and Bit Operations/Compare To Zero  relop=<  OutDataTypeStr=boolean  ZeroCross=off
  Vmin>0 : simulink/Logic and Bit Operations/Compare To Zero  relop=>  OutDataTypeStr=boolean  ZeroCross=off
  Out1 : Outport
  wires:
  Switch2/1 -> Sum1/1
  Switch/1 -> Sum1/2
  Constant1/1 -> Switch1/1, Switch/1, Switch2/1
  Sum1/1 -> Out1/1
  In1/1 -> MinMax1/1, MinMax/1
  Switch1/1 -> Sum1/3
  Sum/1 -> Switch2/3
  Logical Operator2/1 -> Switch2/2
  Vmax<0/1 -> Logical Operator/1, Switch1/2
  Vmin>0/1 -> Logical Operator1/1, Switch/2
  Logical Operator1/1 -> Logical Operator2/2
  Logical Operator/1 -> Logical Operator2/1
  Gain1/1 -> Sum/2, Switch/3, Vmax<0/1
  Gain/1 -> Sum/1, Vmin>0/1, Switch1/3
  MinMax1/1 -> Gain1/1
  MinMax/1 -> Gain/1

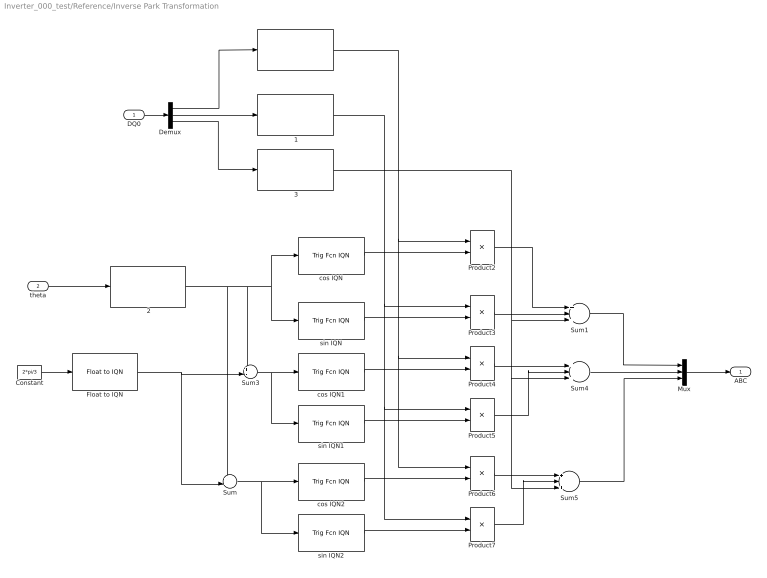
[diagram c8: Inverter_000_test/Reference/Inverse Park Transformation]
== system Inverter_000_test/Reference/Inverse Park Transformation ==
  DQ0 : Inport
  theta : Inport  Port=2
   {,1..3} (4 alike) : etargetslib/ 
  Constant : Constant  Value=2*pi/3  OutDataTypeStr=single
  Demux : Demux  Outputs=3
  Float to IQN : tiiqmathlib/Float to IQN  Q_value=10
  Mux : Mux  Inputs=3
  Product{2..7} (6 alike) : Product
  Sum : Sum  Inputs=++|
  Sum1 : Sum  Inputs=+-+
  Sum3 : Sum  Inputs=+-|
  Sum4 : Sum  Inputs=+-+
  Sum5 : Sum  Inputs=+-+
  cos IQN : tiiqmathlib/Trig Fcn IQN  functionOption=_IQcos
  cos IQN1 : tiiqmathlib/Trig Fcn IQN  functionOption=_IQcos
  cos IQN2 : tiiqmathlib/Trig Fcn IQN  functionOption=_IQcos
  sin IQN : tiiqmathlib/Trig Fcn IQN  functionOption=_IQsin
  sin IQN1 : tiiqmathlib/Trig Fcn IQN  functionOption=_IQsin
  sin IQN2 : tiiqmathlib/Trig Fcn IQN  functionOption=_IQsin
  ABC : Outport
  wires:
  " 2"/1 -> sin IQN/1, cos IQN/1, Sum3/1, Sum/1
  " 1"/1 -> Product7/1, Product5/1, Product3/1
  Product2/1 -> Sum1/1
  Product3/1 -> Sum1/2
  sin IQN/1 -> Product3/2
  cos IQN/1 -> Product2/2
  Demux/2 -> " 1"/1
  Demux/1 -> " "/1
  theta/1 -> " 2"/1
  Demux/3 -> " 3"/1
  Constant/1 -> Float to IQN/1
  Float to IQN/1 -> Sum/2, Sum3/2
  " 3"/1 -> Sum5/3, Sum4/3, Sum1/3
  Sum3/1 -> sin IQN1/1, cos IQN1/1
  cos IQN1/1 -> Product4/2
  sin IQN1/1 -> Product5/2
  Product4/1 -> Sum4/1
  Product5/1 -> Sum4/2
  Sum4/1 -> Mux/2
  Sum/1 -> sin IQN2/1, cos IQN2/1
  " "/1 -> Product2/1, Product4/1, Product6/1
  cos IQN2/1 -> Product6/2
  sin IQN2/1 -> Product7/2
  Product6/1 -> Sum5/1
  Product7/1 -> Sum5/2
  Sum5/1 -> Mux/3
  DQ0/1 -> Demux/1
  Sum1/1 -> Mux/1
  Mux/1 -> ABC/1

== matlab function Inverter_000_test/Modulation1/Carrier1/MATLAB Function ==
function y = fcn(In1, In2)

temp_min = -0.5 * In1; % min
temp_max = -0.5 * In2; % max
temp_mid = temp_min + temp_max; % min

y = temp_mid;

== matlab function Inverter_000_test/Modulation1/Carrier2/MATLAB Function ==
function y = fcn(In1, In2)

temp_min = -0.5 * In1; % min
temp_max = -0.5 * In2; % max
temp_mid = temp_min + temp_max; % min

y = temp_mid;

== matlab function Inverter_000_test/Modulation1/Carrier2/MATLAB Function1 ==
function y = fcn(In1, In2)

temp_min = -0.5 * In1; % min
temp_max = -0.5 * In2; % max
temp_mid = temp_min + temp_max; % min

if temp_min > 0 
    temp_out1 = temp_max * 0.0;
else
    temp_out1 = temp_max;
end
if temp_max < 0
    temp_out2 = temp_min * 0.0;
else
    temp_out2 = temp_min;
end
if ~(temp_min > 0) && ~(temp_max < 0)
    temp_out3 = temp_mid * 0.0;
else
    temp_out3 = temp_mid;
end

temp_out = temp_out1 + temp_out2 + temp_out3;

y = temp_out;
